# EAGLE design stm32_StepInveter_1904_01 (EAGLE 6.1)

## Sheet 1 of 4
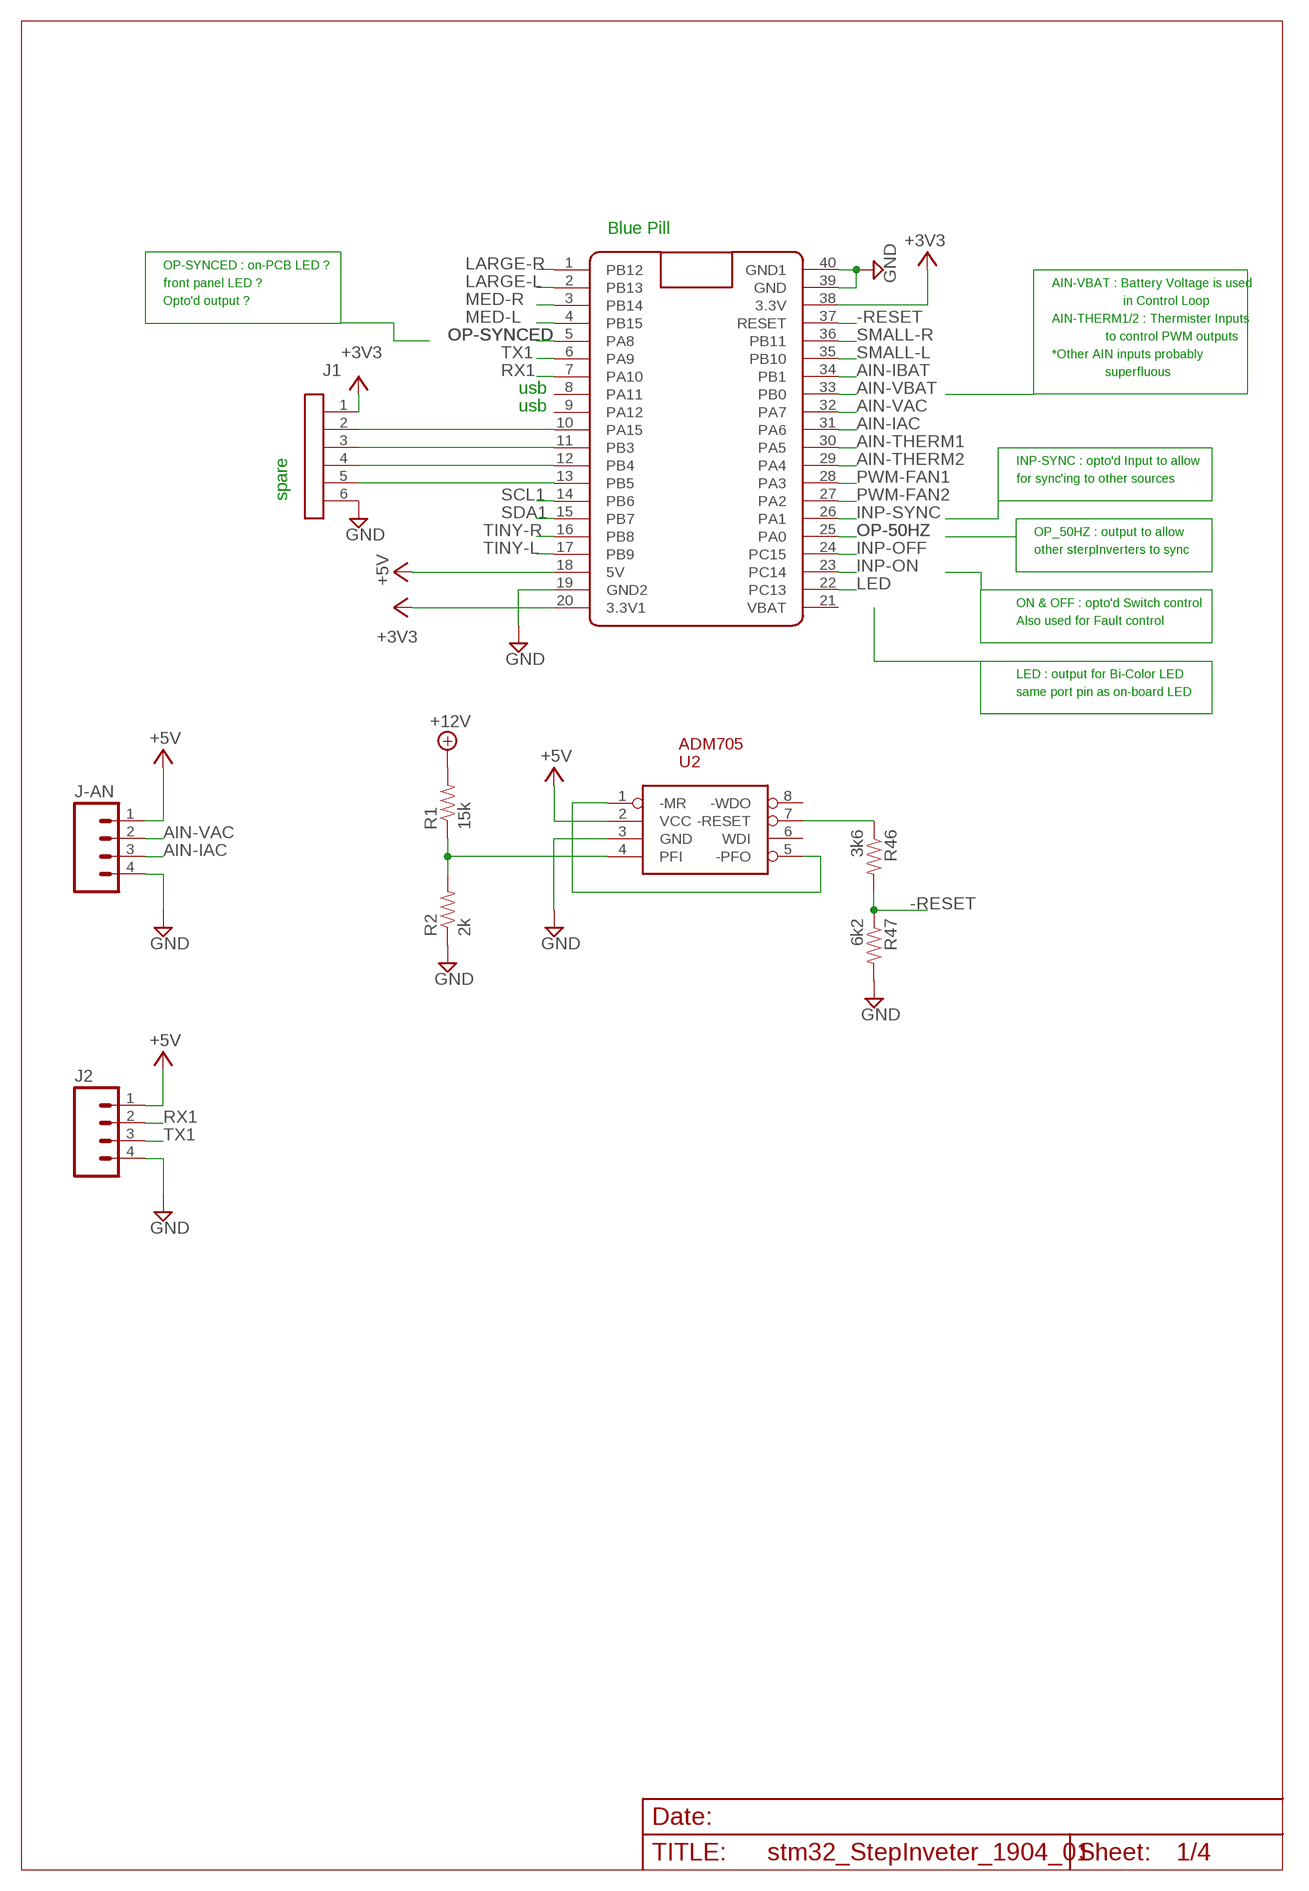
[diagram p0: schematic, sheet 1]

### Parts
J1  SIL-6  [SIL6]
J2  SIL4  [SIL4]
J-AN  SIL4  [SIL4]
R1  15k  R4  [AXIAL-0.4]
R2  2k  R4  [AXIAL-0.4]
R46  3k6  R4  [AXIAL-0.4]
R47  6k2  R4  [AXIAL-0.4]
U2  ADM705  [DIL08]
U$1  BLUE_PILL  [BLUE_PILL_CLEAN]

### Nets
+3V3: J1.1 U$1.20(3.3V1) U$1.38(3.3V) ; also sheet 3
+5V: J2.1 J-AN.1 U2.2(VCC) U$1.18(5V) ; also sheet 2,3,4
+12V: R1.P$2 ; also sheet 3
-RESET: R46.P$2 R47.P$1 U$1.37(RESET)
AIN-IAC: J-AN.3 U$1.31(PA6)
AIN-IBAT: U$1.34(PB1) ; also sheet 3
AIN-THERM1: U$1.30(PA5) ; also sheet 3
AIN-THERM2: U$1.29(PA4) ; also sheet 3
AIN-VAC: J-AN.2 U$1.32(PA7)
AIN-VBAT: U$1.33(PB0) ; also sheet 3
GND: J1.6 J2.4 J-AN.4 R2.P$1 R47.P$2 U2.3(GND) U$1.19(GND2) U$1.39(GND) U$1.40(GND1) ; also sheet 2,3,4
INP-OFF: U$1.24(PC15) ; also sheet 3
INP-ON: U$1.23(PC14) ; also sheet 3
INP-SYNC: U$1.26(PA1) ; also sheet 3
LARGE-L: U$1.2(PB13) ; also sheet 2
LARGE-R: U$1.1(PB12) ; also sheet 2
LED: U$1.22(PC13) ; also sheet 4
MED-L: U$1.4(PB15) ; also sheet 2
MED-R: U$1.3(PB14) ; also sheet 2
N$1: J1.2 U$1.10(PA15)
N$2: J1.3 U$1.11(PB3)
N$3: J1.4 U$1.12(PB4)
N$4: J1.5 U$1.13(PB5)
N$5: U2.1(-MR) U2.5(-PFO)
N$6: R1.P$1 R2.P$2 U2.4(PFI)
N$77: R46.P$1 U2.7(-RESET)
OP-50HZ: U$1.25(PA0) ; also sheet 4
OP-SYNCED: U$1.5(PA8) ; also sheet 4
PWM-FAN1: U$1.28(PA3) ; also sheet 4
PWM-FAN2: U$1.27(PA2) ; also sheet 4
RX1: J2.2 U$1.7(PA10)
SCL1: U$1.14(PB6)
SDA1: U$1.15(PB7)
SMALL-L: U$1.35(PB10) ; also sheet 2
SMALL-R: U$1.36(PB11) ; also sheet 2
TINY-L: U$1.17(PB9) ; also sheet 2
TINY-R: U$1.16(PB8) ; also sheet 2
TX1: J2.3 U$1.6(PA9)
Unconnected: U2.6(WDI) U2.8(-WDO) U$1.8(PA11) U$1.9(PA12) U$1.21(VBAT)

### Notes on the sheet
- Blue Pill
- OP-SYNCED : on-PCB LED ?
- front panel LED ? | AIN-VBAT : Battery Voltage is used
- Opto'd output ? | in Control Loop
- AIN-THERM1/2 : Thermister Inputs
- to control PWM outputs
- *Other AIN inputs probably
- superfluous
- usb
- usb
- INP-SYNC : opto'd Input to allow
- for sync'ing to other sources
- spare
- OP_50HZ : output to allow
- other sterpInverters to sync
- ON & OFF : opto'd Switch control
- Also used for Fault control
- LED : output for Bi-Color LED
- same port pin as on-board LED

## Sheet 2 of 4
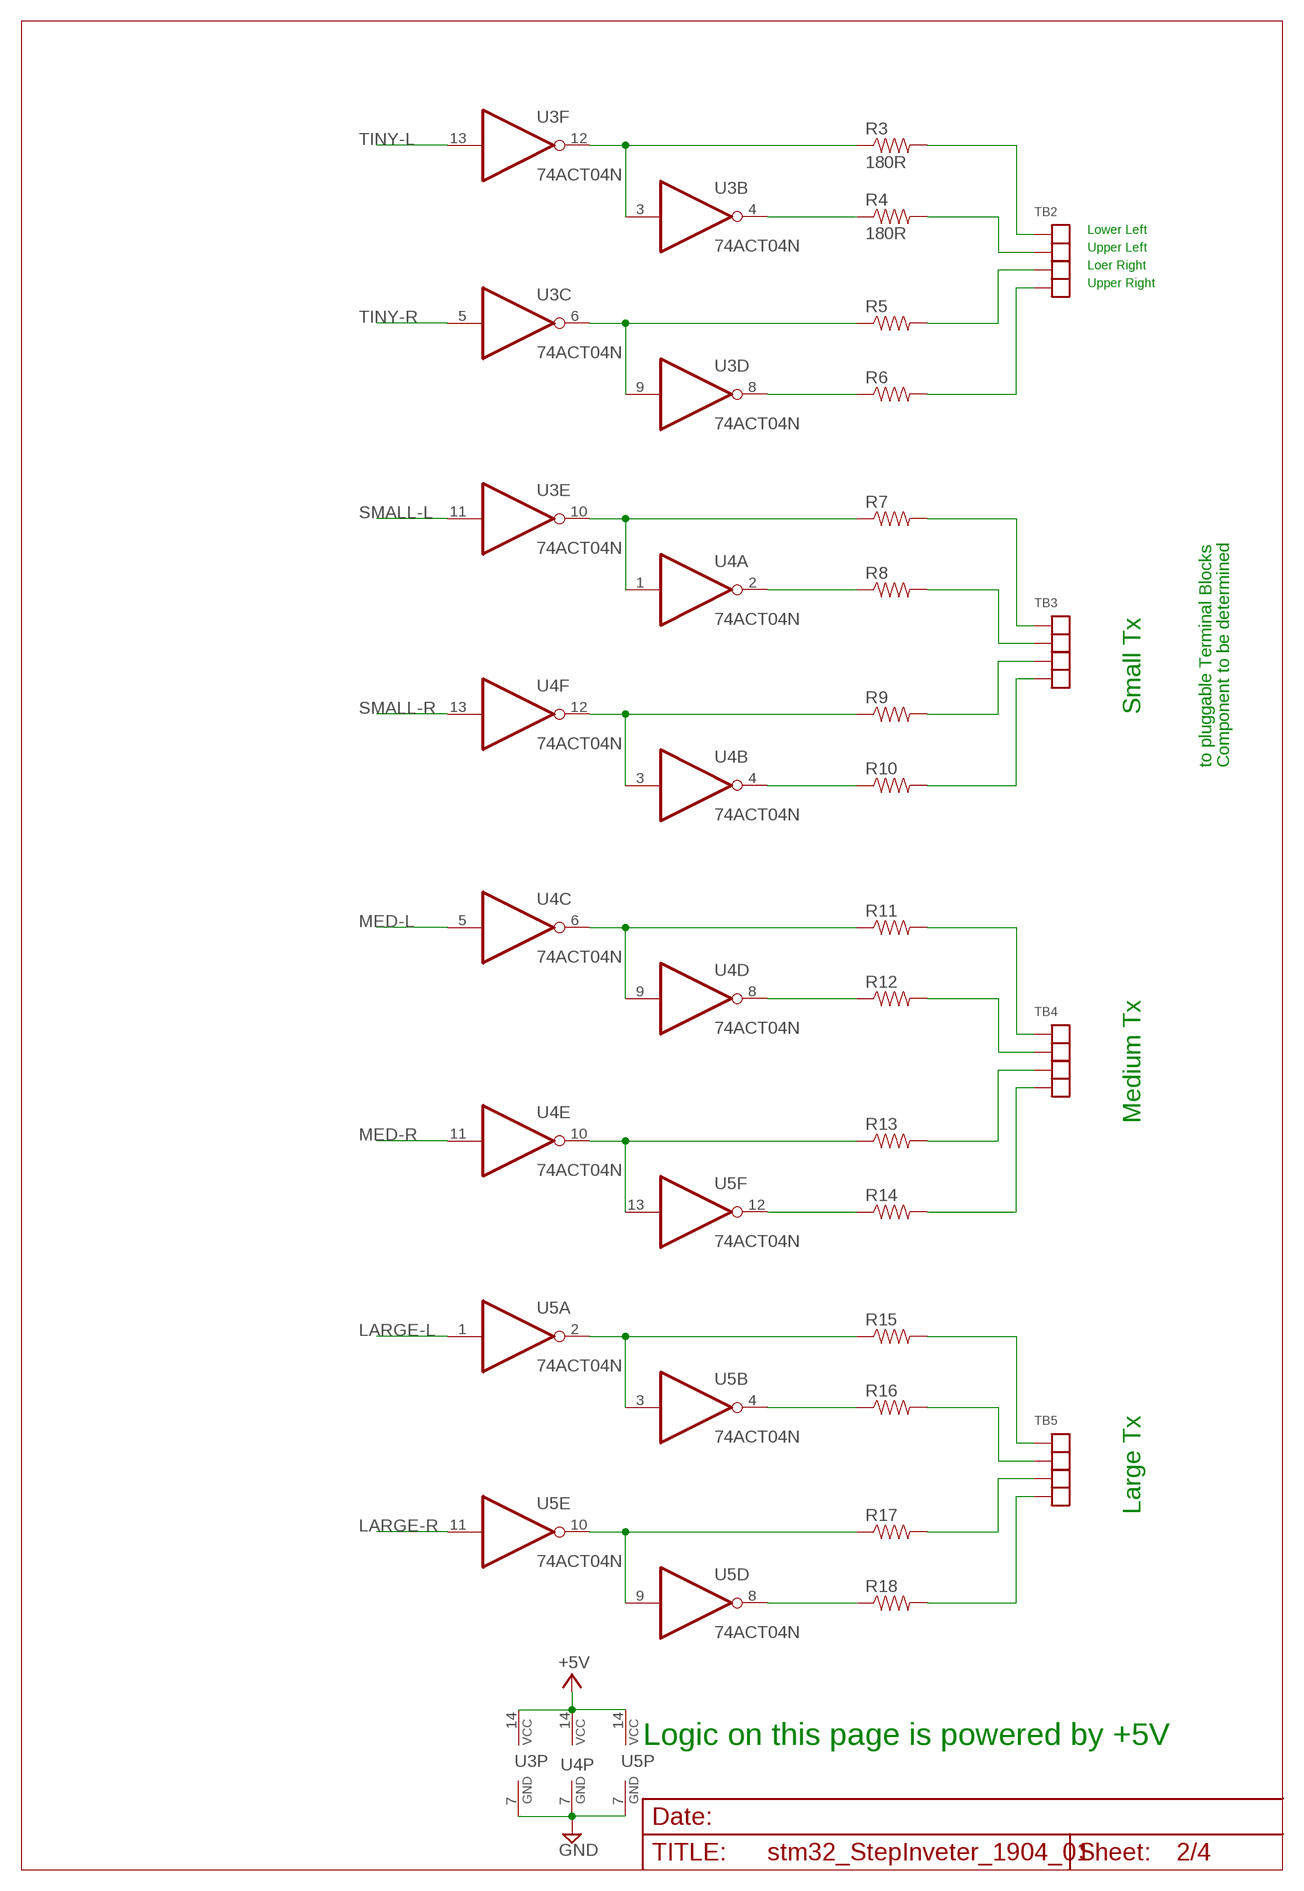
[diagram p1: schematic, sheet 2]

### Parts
R3  180R  R4  [AXIAL-0.4]
R4  180R  R4  [AXIAL-0.4]
R5  R4  [AXIAL-0.4]
R6  R4  [AXIAL-0.4]
R7  R4  [AXIAL-0.4]
R8  R4  [AXIAL-0.4]
R9  R4  [AXIAL-0.4]
R10  R4  [AXIAL-0.4]
R11  R4  [AXIAL-0.4]
R12  R4  [AXIAL-0.4]
R13  R4  [AXIAL-0.4]
R14  R4  [AXIAL-0.4]
R15  R4  [AXIAL-0.4]
R16  R4  [AXIAL-0.4]
R17  R4  [AXIAL-0.4]
R18  R4  [AXIAL-0.4]
TB2  TB4381_SIL  [TB-381-SIL-4P]
TB3  TB4381_SIL  [TB-381-SIL-4P]
TB4  TB4381_SIL  [TB-381-SIL-4P]
TB5  TB4381_SIL  [TB-381-SIL-4P]
U3  74ACT04N  [DIL14]
U4  74ACT04N  [DIL14]
U5  74ACT04N  [DIL14]

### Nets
+5V: U3.14(P:VCC) U4.14(P:VCC) U5.14(P:VCC) ; also sheet 1,3,4
GND: U3.7(P:GND) U4.7(P:GND) U5.7(P:GND) ; also sheet 1,3,4
LARGE-L: U5.1(A:I) ; also sheet 1
LARGE-R: U5.11(E:I) ; also sheet 1
MED-L: U4.5(C:I) ; also sheet 1
MED-R: U4.11(E:I) ; also sheet 1
N$15: R3.P$1 U3.3(B:I) U3.12(F:O)
N$16: R4.P$1 U3.4(B:O)
N$17: R5.P$1 U3.6(C:O) U3.9(D:I)
N$18: R6.P$1 U3.8(D:O)
N$19: R7.P$1 U3.10(E:O) U4.1(A:I)
N$20: R8.P$1 U4.2(A:O)
N$21: R9.P$1 U4.3(B:I) U4.12(F:O)
N$22: R10.P$1 U4.4(B:O)
N$23: R11.P$1 U4.6(C:O) U4.9(D:I)
N$24: R12.P$1 U4.8(D:O)
N$25: R13.P$1 U4.10(E:O) U5.13(F:I)
N$26: R14.P$1 U5.12(F:O)
N$27: R15.P$1 U5.2(A:O) U5.3(B:I)
N$28: R16.P$1 U5.4(B:O)
N$29: R17.P$1 U5.9(D:I) U5.10(E:O)
N$30: R18.P$1 U5.8(D:O)
N$40: R3.P$2 TB2.1 TB2.11
N$62: R4.P$2 TB2.2 TB2.12
N$63: R5.P$2 TB2.3 TB2.13
N$64: R6.P$2 TB2.4 TB2.14
N$65: R7.P$2 TB3.1 TB3.11
N$66: R8.P$2 TB3.2 TB3.12
N$67: R9.P$2 TB3.3 TB3.13
N$68: R10.P$2 TB3.4 TB3.14
N$69: R11.P$2 TB4.1 TB4.11
N$70: R12.P$2 TB4.2 TB4.12
N$71: R13.P$2 TB4.3 TB4.13
N$72: R14.P$2 TB4.4 TB4.14
N$73: R15.P$2 TB5.1 TB5.11
N$74: R16.P$2 TB5.2 TB5.12
N$75: R17.P$2 TB5.3 TB5.13
N$76: R18.P$2 TB5.4 TB5.14
SMALL-L: U3.11(E:I) ; also sheet 1
SMALL-R: U4.13(F:I) ; also sheet 1
TINY-L: U3.13(F:I) ; also sheet 1
TINY-R: U3.5(C:I) ; also sheet 1

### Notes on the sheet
- Lower Left
- Upper Left
- Loer Right
- Upper Right
- Small Tx
- to pluggable Terminal Blocks | Component to be determined
- Medium Tx
- Large Tx
- Logic on this page is powered by +5V

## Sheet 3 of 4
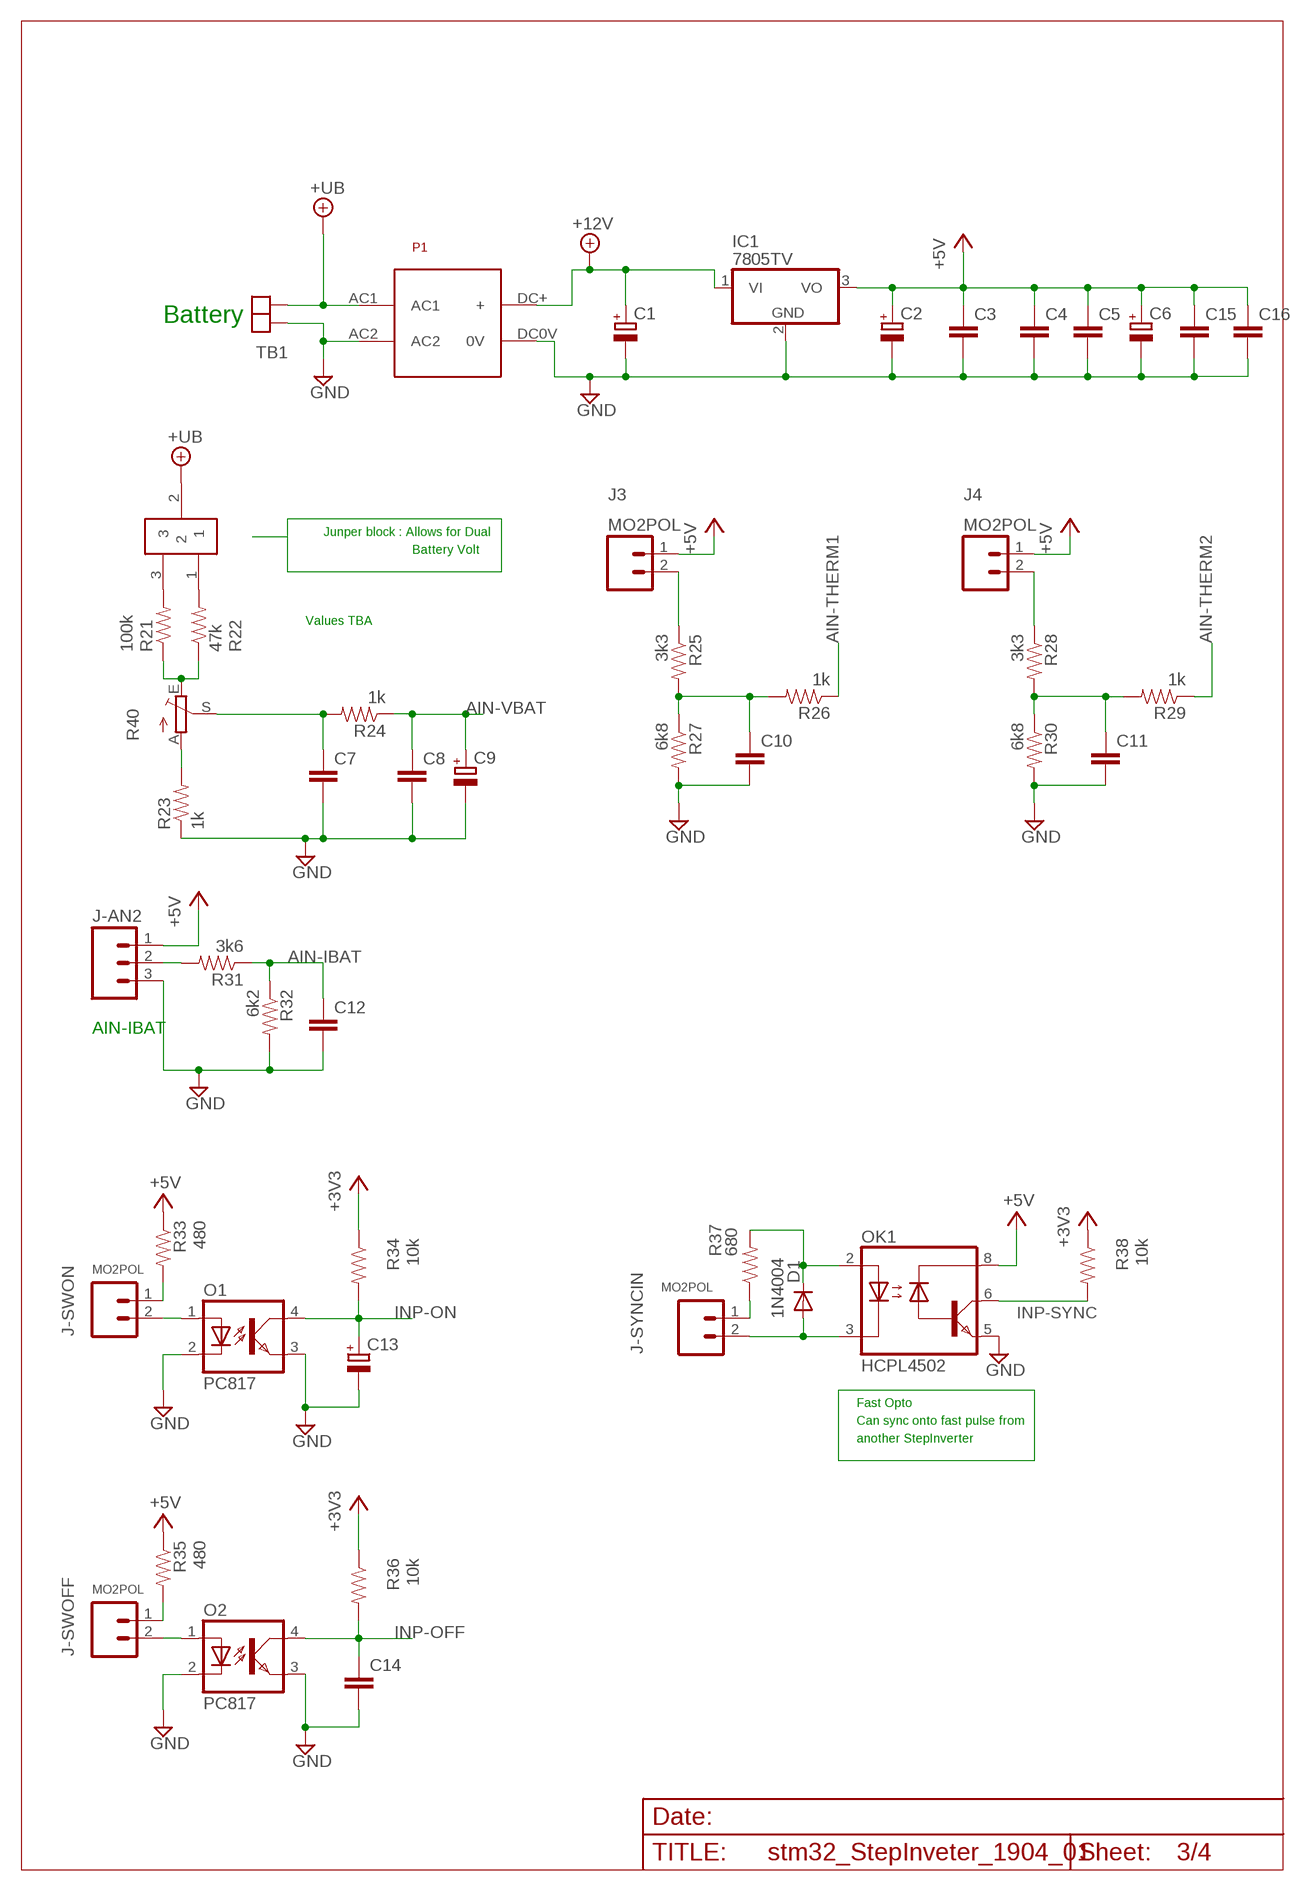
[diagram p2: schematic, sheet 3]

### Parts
C1  CPOL-EUE5-8.5  [E5-8,5]
C2  CPOL-EUE2.5-5  [E2,5-5]
C3  BCAP  [BCAP]
C4  BCAP  [BCAP]
C5  BCAP  [BCAP]
C6  CPOL-EUE2.5-5  [E2,5-5]
C7  BCAP  [BCAP]
C8  BCAP  [BCAP]
C9  CPOL-EUE2.5-5  [E2,5-5]
C10  BCAP  [BCAP]
C11  BCAP  [BCAP]
C12  BCAP  [BCAP]
C13  CPOL-EUE2.5-6  [E2,5-6]
C14  BCAP  [BCAP]
C15  BCAP  [BCAP]
C16  BCAP  [BCAP]
D1  1N4004  [DO41-10]
IC1  7805TV  [TO220V]
J3  MO2POL  [MOLEX-1X2]
J4  MO2POL  [MOLEX-1X2]
J-AN2  MO3POL  [MOLEX-3]
J-SWOFF  MO2POL  [MOLEX-1X2]
J-SWON  MO2POL  [MOLEX-1X2]
J-SYNCIN  MO2POL  [MOLEX-1X2]
JP1  JP1X3  [JP1X3]
O1  PC817  [DIL04]
O2  PC817  [DIL04]
OK1  HCPL4502  [DIL08]
P1  ACDC  [ACDC]
R21  100k  R4  [AXIAL-0.4]
R22  47k  R4  [AXIAL-0.4]
R23  1k  R4  [AXIAL-0.4]
R24  1k  R4  [AXIAL-0.4]
R25  3k3  R4  [AXIAL-0.4]
R26  1k  R4  [AXIAL-0.4]
R27  6k8  R4  [AXIAL-0.4]
R28  3k3  R4  [AXIAL-0.4]
R29  1k  R4  [AXIAL-0.4]
R30  6k8  R4  [AXIAL-0.4]
R31  3k6  R4  [AXIAL-0.4]
R32  6k2  R4  [AXIAL-0.4]
R33  480  R4  [AXIAL-0.4]
R34  10k  R4  [AXIAL-0.4]
R35  480  R4  [AXIAL-0.4]
R36  10k  R4  [AXIAL-0.4]
R37  680  R4  [AXIAL-0.4]
R38  10k  R4  [AXIAL-0.4]
R40  TRIM_EU-B64Y  [B64Y]
TB1  TB2381  [TB-KF2EDG381-2P]

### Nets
+3V3: R34.P$1 R36.P$1 R38.P$1 ; also sheet 1
+5V: C2.+ C3.1 C4.1 C5.1 C6.+ C15.1 C16.1 IC1.3(VO) J3.1 J4.1 J-AN2.1 OK1.8(VCC) R33.P$1 R35.P$1 ; also sheet 1,2,4
+12V: C1.+ IC1.1(VI) P1.DC+(+) ; also sheet 1
+UB: JP1.2 P1.AC1 TB1.1
AIN-IBAT: C12.1 R31.P$1 R32.P$1 ; also sheet 1
AIN-THERM1: R26.P$1 ; also sheet 1
AIN-THERM2: R29.P$1 ; also sheet 1
AIN-VBAT: C8.1 C9.+ R24.P$1 ; also sheet 1
GND: C1.- C2.- C3.2 C4.2 C5.2 C6.- C7.2 C8.2 C9.- C10.2 C11.2 C12.2 C13.- C14.2 C15.2 C16.2 IC1.2(GND) J-AN2.3 O1.2(C) O1.3(EMIT) O2.2(C) O2.3(EMIT) OK1.5(GND) P1.AC2 P1.DC0V(0V) R23.P$1 R27.P$2 R30.P$2 R32.P$2 TB1.2 ; also sheet 1,2,4
INP-OFF: C14.1 O2.4(COL) R36.P$2 ; also sheet 1
INP-ON: C13.+ O1.4(COL) R34.P$2 ; also sheet 1
INP-SYNC: OK1.6(VO) R38.P$2 ; also sheet 1
N$14: JP1.3 R21.P$2
N$32: JP1.1 R22.P$2
N$34: R21.P$1 R22.P$1 R40.E
N$35: C10.1 R25.P$2 R26.P$2 R27.P$1
N$36: J4.2 R28.P$1
N$37: J3.2 R25.P$1
N$38: C11.1 R28.P$2 R29.P$2 R30.P$1
N$39: J-SWON.1 R33.P$2
N$41: J-AN2.2 R31.P$2
N$42: J-SWON.2 O1.1(A)
N$43: J-SYNCIN.1 R37.P$1
N$44: D1.A J-SYNCIN.2 OK1.3(C)
N$45: J-SWOFF.1 R35.P$2
N$46: J-SWOFF.2 O2.1(A)
N$47: D1.C OK1.2(A) R37.P$2
N$82: C7.1 R24.P$2 R40.S
N$84: R23.P$2 R40.A

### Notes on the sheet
- Battery
- Junper block : Allows for Dual
- Battery Volt
- Values TBA
- AIN-IBAT
- Fast Opto
- Can sync onto fast pulse from
- another StepInverter

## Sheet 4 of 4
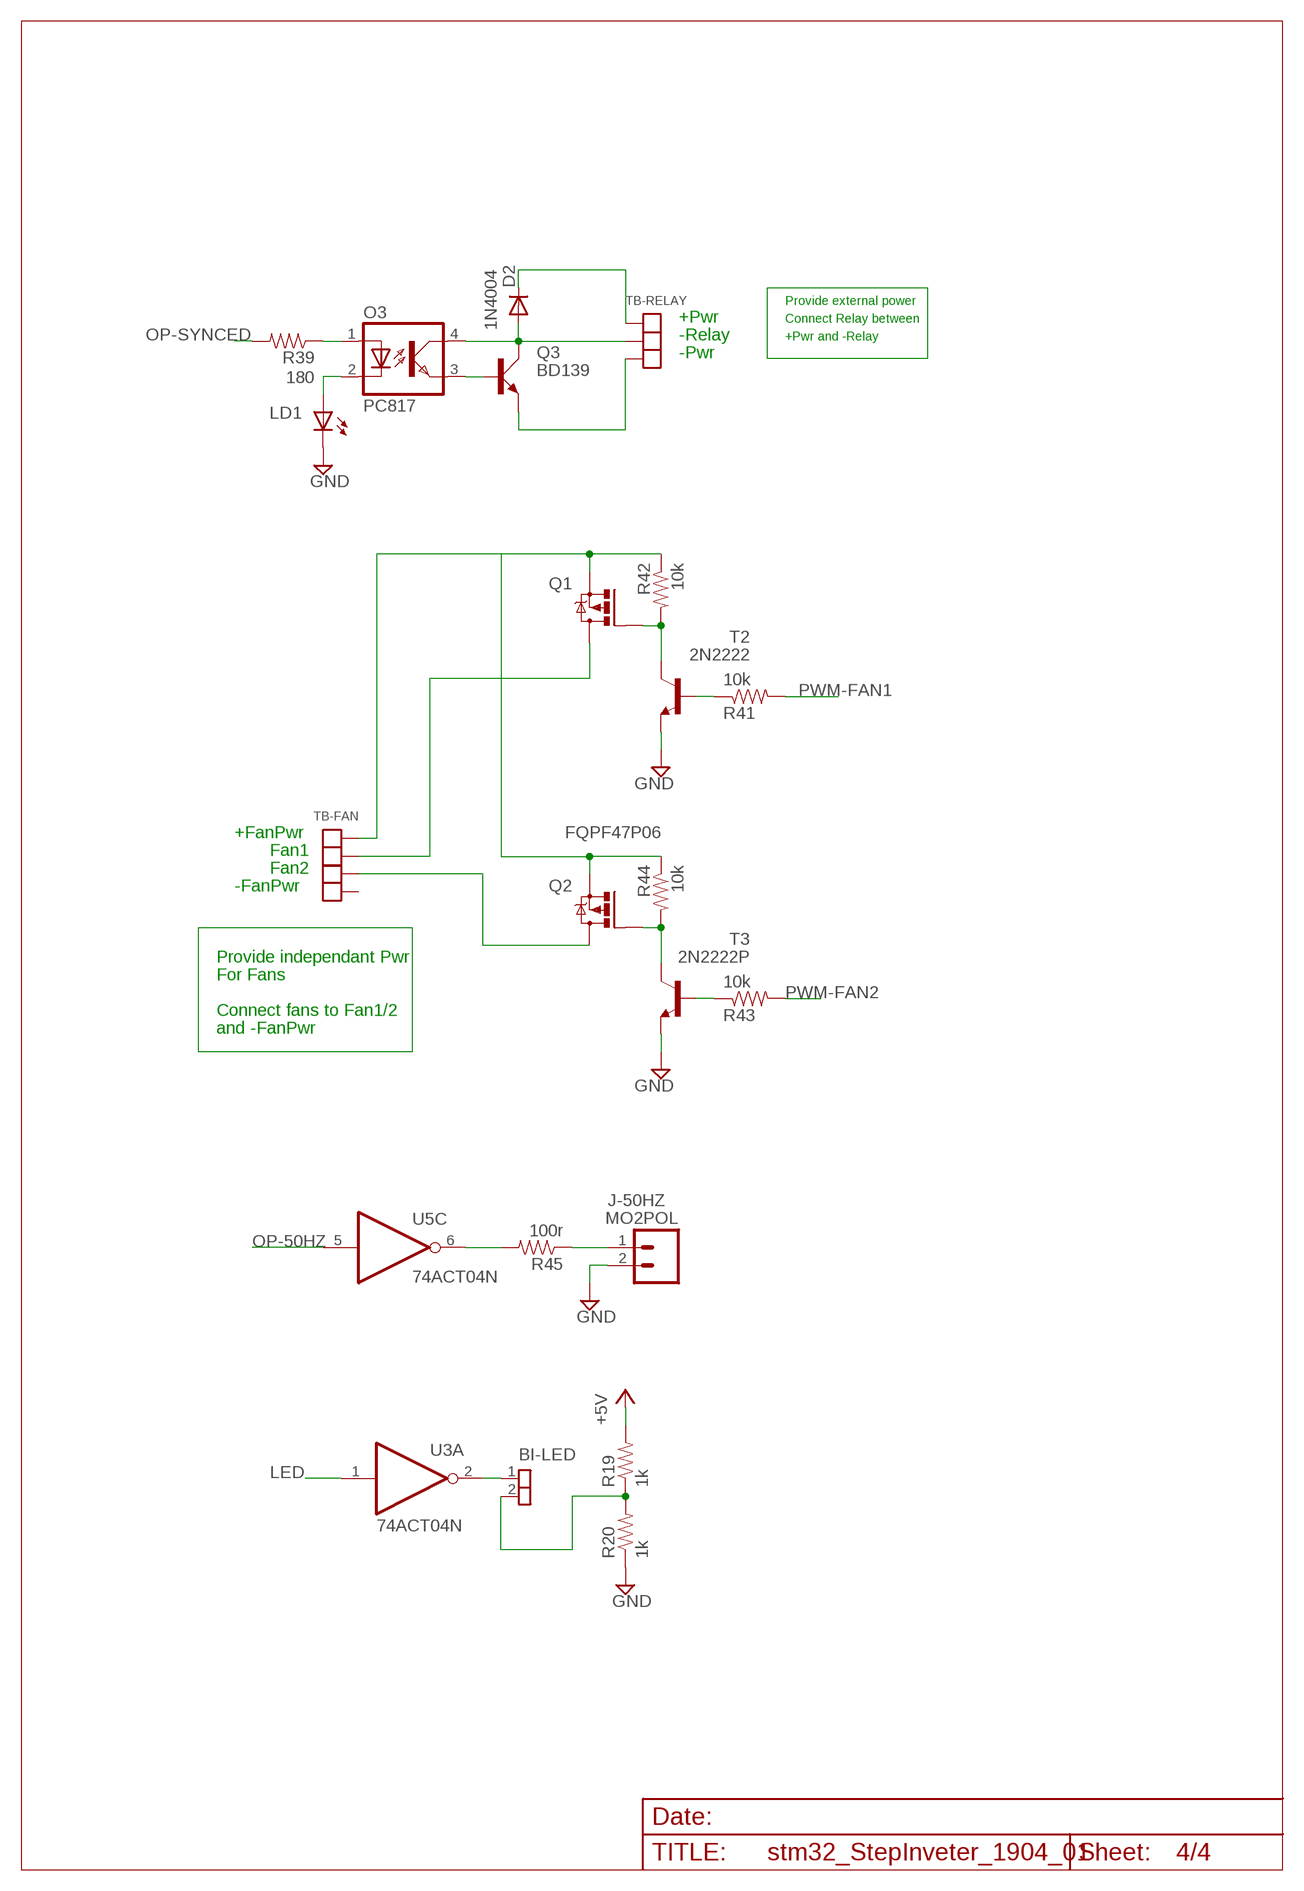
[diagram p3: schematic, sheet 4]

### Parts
BI-LED  SIL-2  [JP1]
D2  1N4004  [DO41-10]
J-50HZ  MO2POL  [MOLEX-1X2]
LD1  LED3MM  [LED3MM]
O3  PC817  [DIL04]
Q1  MOSFET-PCHFQPF47P06  [TO220BV]
Q2  FQPF47P06  MOSFET-PCHFQPF47P06  [TO220BV]
Q3  BD139  [TO126AV]
R19  1k  R4  [AXIAL-0.4]
R20  1k  R4  [AXIAL-0.4]
R39  180  R4  [AXIAL-0.4]
R41  10k  R4  [AXIAL-0.4]
R42  10k  R4  [AXIAL-0.4]
R43  10k  R4  [AXIAL-0.4]
R44  10k  R4  [AXIAL-0.4]
R45  100r  R4  [AXIAL-0.4]
T2  2N2222  2N2222P  [TO92/]
T3  2N2222P  [TO92/]
TB-FAN  TB4  [TB-KF2EDG381-4P]
TB-RELAY  TB3381  [TB-KF2EDG381-3P]

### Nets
+5V: R19.P$2 ; also sheet 1,2,3
GND: J-50HZ.2 LD1.K(C) R20.P$1 T2.1(E) T3.1(E) ; also sheet 1,2,3
LED: U3.1(A:I) ; also sheet 1
N$7: BI-LED.2 R19.P$1 R20.P$2
N$8: BI-LED.1 U3.2(A:O)
N$49: LD1.A O3.2(C)
N$50: O3.1(A) R39.P$1
N$51: Q1.G R42.P$2 T2.3(C)
N$52: O3.3(EMIT) Q3.B
N$53: R41.P$1 T2.2(B)
N$54: Q1.S Q2.S R42.P$1 R44.P$1 TB-FAN.1
N$55: Q2.G R44.P$2 T3.3(C)
N$56: R45.P$2 U5.6(C:O)
N$57: Q1.D TB-FAN.2
N$58: R43.P$1 T3.2(B)
N$59: J-50HZ.1 R45.P$1
N$60: Q2.D TB-FAN.3
N$78: D2.A O3.4(COL) Q3.C TB-RELAY.2
N$79: D2.C TB-RELAY.1
N$81: Q3.E TB-RELAY.3
OP-50HZ: U5.5(C:I) ; also sheet 1
OP-SYNCED: R39.P$2 ; also sheet 1
PWM-FAN1: R41.P$2 ; also sheet 1
PWM-FAN2: R43.P$2 ; also sheet 1
Unconnected: TB-FAN.4

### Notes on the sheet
- Provide external power
- +Pwr | Connect Relay between
- -Relay | +Pwr and -Relay
- -Pwr
- +FanPwr
- Fan1
- Fan2
- -FanPwr
- Provide independant Pwr
- For Fans
- Connect fans to Fan1/2
- and -FanPwr

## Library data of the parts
BI-LED = Andrew_Connectors:SIL-2
C1 C2 C6 C9 C13 = rcl:CPOL-EU: POLARIZED CAPACITOR, European symbol
C3-C5 C7 C8 C10-C12 C14-C16 = Andrew Misc:BCAP
D1 D2 = diode:1N4004: DIODE
IC1 = Andrew Linear:78*: Positive VOLTAGE REGULATOR Source: http://cache.national.com/ds/LM/LM78L05.pdf http://www.fairchildsemi.com/ds/LM/LM7805.pdf
J1 = Andrew_Connectors:SIL-6
J2 J-AN = Andrew_Connectors:SIL4
J3 J4 J-50HZ J-SWOFF J-SWON J-SYNCIN = Andrew_Connectors:MO2POL
J-AN2 = Andrew_Connectors:MO3POL
JP1 = Andrew_Connectors:JP1X3
LD1 = led:LED: LED
O1-O3 = Andrew:PC817: SHARP OPTO COUPLER; MPN: PC817X4J000F; OC_FARNELL: 9707727; OC_NEWARK: 97K7059
OK1 = optocoupler:HCPL4502: HEWLETT PACKARD OPTO COUPLER; MF: AGILENT TECHNOLOGIES; MPN: HCPL-4502-000E; OC_FARNELL: 9994777; OC_NEWARK: 31K7017
P1 = Andrew ISOPWR:ACDC
Q1 Q2 = Andrew Transistor:MOSFET-PCH: P-CHANNEL HEXFET POWER-MOS-FET Source: http://www.irf.com/product-info/datasheets/data/irf9530.pdf
Q3 = transistor-power:BD139: NPN TRANSISTOR
R1-R39 R41-R47 = Andrew Misc:R4
R40 = pot:TRIM_EU-: POTENTIOMETER
T2 T3 = Andrew Transistor:2N2222: NPN TRANSISTOR
TB1 = Andrew_Connectors:TB2
TB2-TB5 TB-FAN = Andrew_Connectors:TB4
TB-RELAY = Andrew_Connectors:TB3
U2 = Andrew IC:ADM705
U3-U5 = 74xx-eu:74*04: Hex INVERTER
U$1 = Andrew_BluePill_Scope:BLUE_PILL

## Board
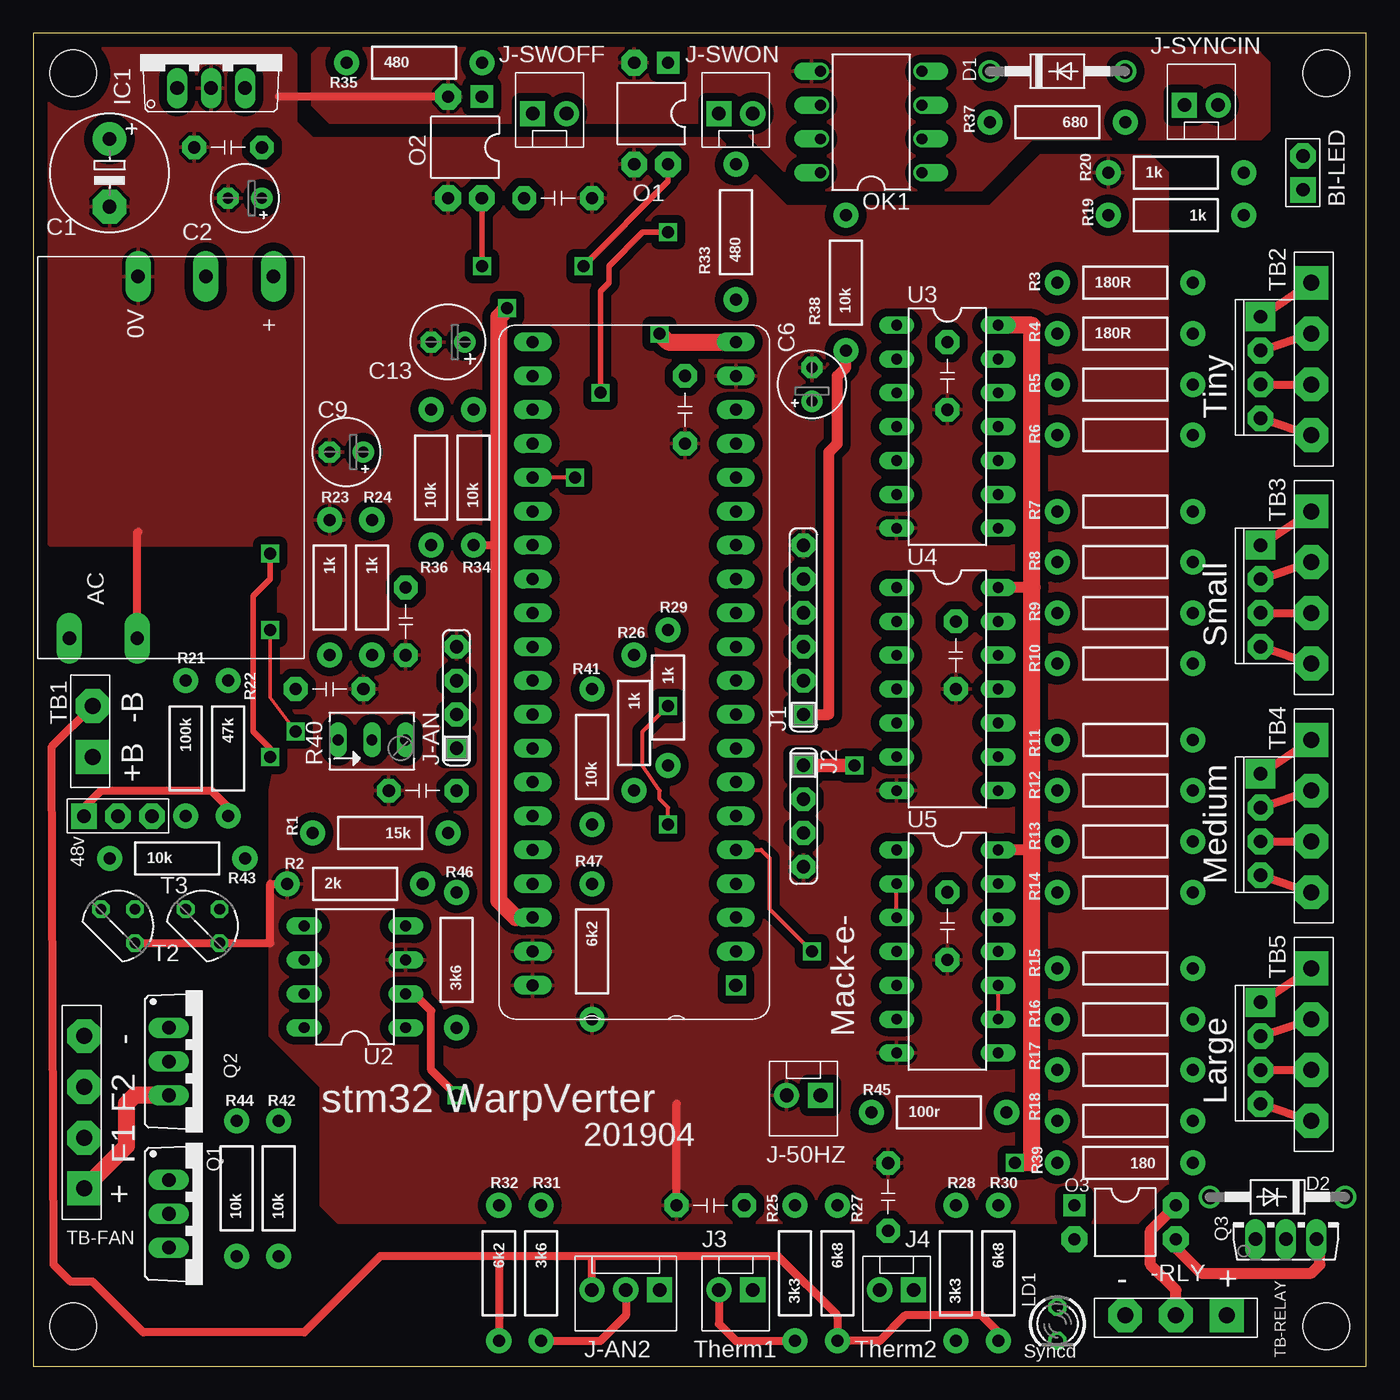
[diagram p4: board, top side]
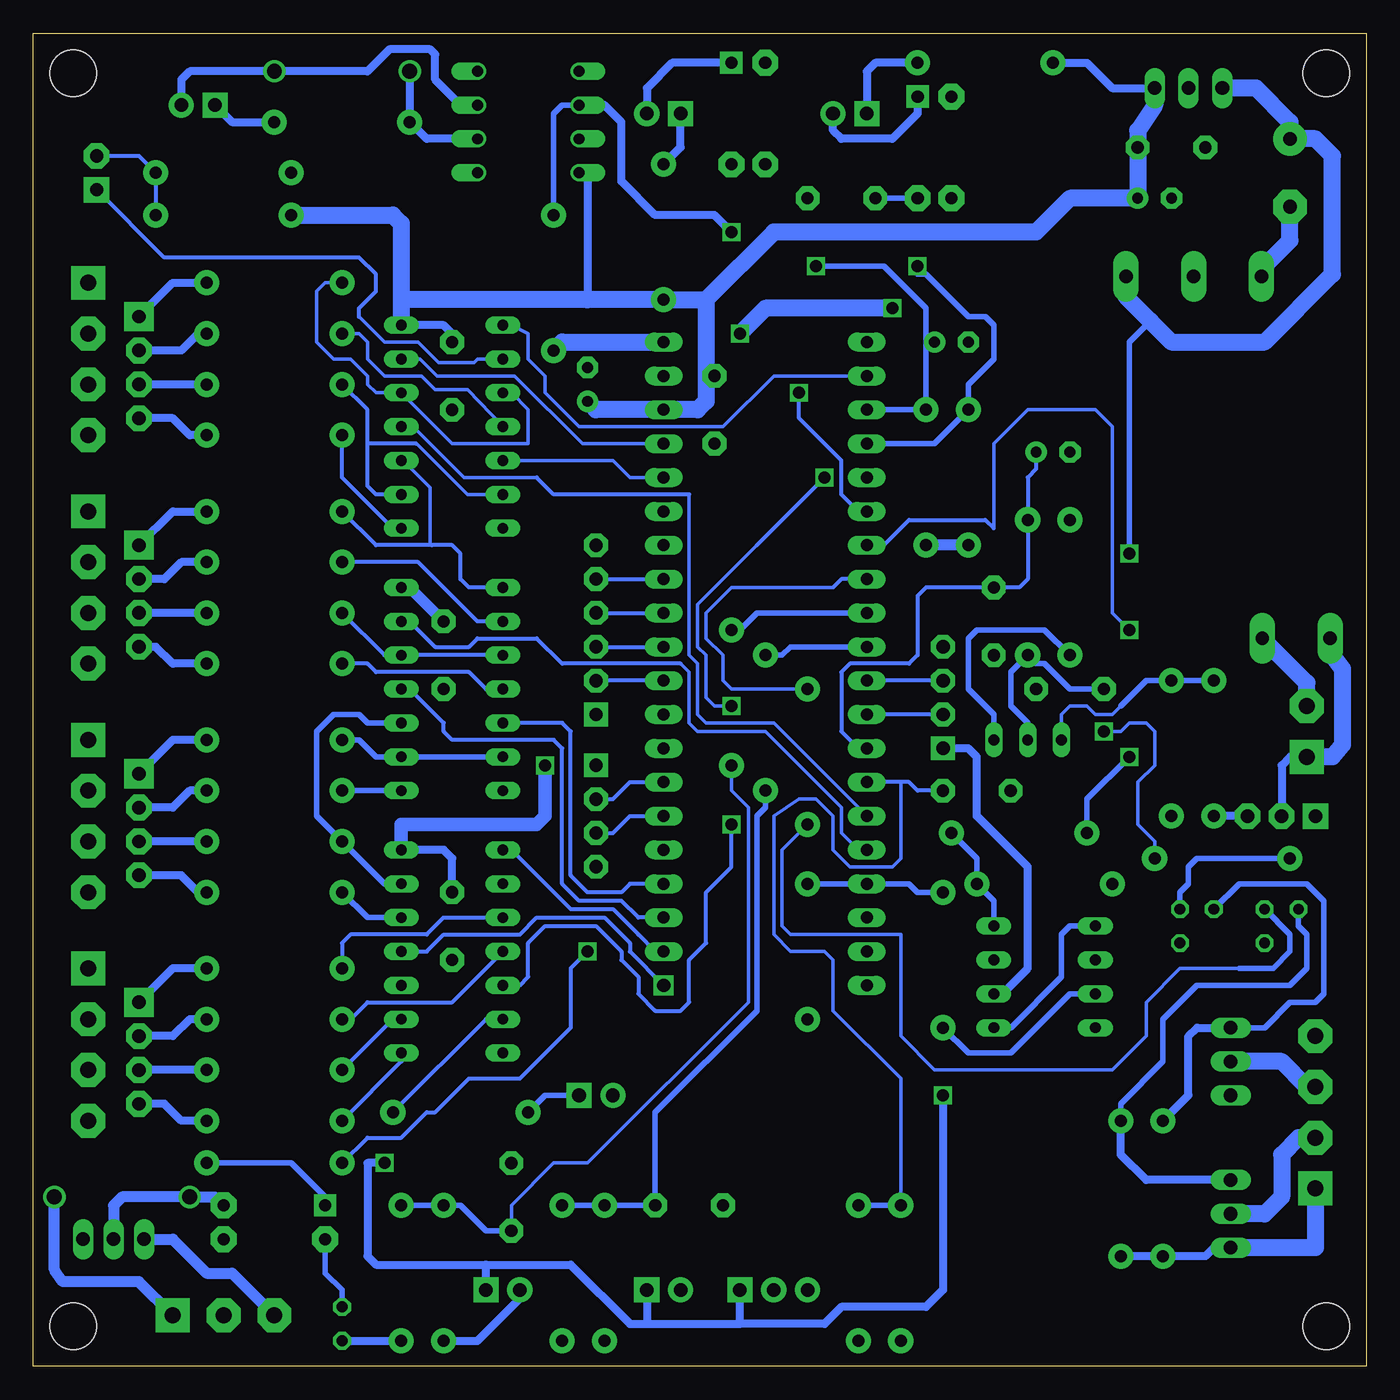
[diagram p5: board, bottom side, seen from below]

Size 100 x 100 mm. Coordinates in mm from the lower left corner, seen from the top.
Outline: 0,0 100,0 100,100 0,100 0,0
Copper layers (1*16): Top 0.035mm / dielectric 1.5mm / Bottom 0.035mm
Design rules: minimum track width 10mil, minimum drill 24mil, track to track 8mil, track to pad 8mil, pad to pad 8mil, via to via 8mil, smd to smd 8mil, copper to edge 40mil, drill to drill 8mil, minimum pad ring 10mil, minimum via ring 8mil, stop-mask expansion 4mil, vias tented up to drill 0mil, thermal gap 10mil
Holes 3.5 mm at 3,3 3,97 97,97 97,3

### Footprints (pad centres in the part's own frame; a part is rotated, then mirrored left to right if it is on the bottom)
JP1 = drill 1 pad 1.905 square: 1 -1.27,0 | drill 1 pad 1.905 octagon: 2 1.27,0
E5-8,5 = drill 1.016 pad 2.54: + -2.54,0 | drill 1.016 pad 2.54 octagon: - 2.54,0
E2,5-5 = drill 0.813 pad 1.6: + -1.27,0 | drill 0.813 pad 1.6 octagon: - 1.27,0
BCAP = drill 0.914 pad 1.778 octagon: 1 -2.54,0; 2 2.54,0
E2,5-6 = drill 0.813 pad 1.6: + -1.27,0 | drill 0.813 pad 1.6 octagon: - 1.27,0
DO41-10 = drill 1.118: A 5.08,0; C -5.08,0
TO220V = drill 1.016 long: 1 -2.54,-2.54; 2 0,-2.54; 3 2.54,-2.54
SIL6 = drill 1 pad 1.778 square: 1 -6.35,0 | drill 1 pad 1.778 octagon: 2 -3.81,0; 3 -1.27,0; 4 1.27,0; 5 3.81,0; 6 6.35,0
SIL4 = drill 1 pad 1.778 square: 1 0,0 | drill 1 pad 1.778 octagon: 2 2.54,0; 3 5.08,0; 4 7.62,0
MOLEX-1X2 = drill 1.016 pad 1.88 square: 1 0,0 | drill 1.016 pad 1.88: 2 2.54,0
MOLEX-3 = drill 1.016 pad 1.88 square: 1 -2.54,0 | drill 1.016 pad 1.88: 2 0,0; 3 2.54,0
JP1X3 = drill 1 pad 1.905 square: 1 -2.54,0 | drill 1 pad 1.905 octagon: 2 0,0; 3 2.54,0
LED3MM = drill 0.813 octagon: A -1.27,0; K 1.27,0
DIL04 = drill 0.914 pad 1.676 square: 1 -1.27,-3.81 | drill 0.914 pad 1.93 octagon: 2 1.27,-3.81; 3 1.27,3.81; 4 -1.27,3.81
DIL08 = drill 0.813 offset: 1 -3.81,-3.81; 2 -1.27,-3.81; 3 1.27,-3.81; 4 3.81,-3.81; 5 3.81,3.81; 6 1.27,3.81; 7 -1.27,3.81; 8 -3.81,3.81
ACDC = drill 1 pad 1.93 long: 4 27.15,7.38; AC1 0,17.61; AC2 0,12.53; DC0V 27.15,12.46; DC+ 27.15,2.3
TO220BV = drill 1.016 long: D 0,-2.54; G -2.54,-2.54; S 2.54,-2.54
TO126AV = drill 1.016 long: B 2.286,-1.27; C 0,-1.27; E -2.286,-1.27
AXIAL-0.4 = drill 0.9 pad 1.88: P$1 -5.08,0; P$2 5.08,0
B64Y = drill 0.813 long: A 2.54,0; E -2.54,0; S 0,0
TO92/ = drill 0.813 octagon: 1 1.27,-1.27; 2 1.27,1.27; 3 -1.27,1.27
TB-KF2EDG381-2P = drill 1.2 pad 2.54 square: 1 0,0 | drill 1.2 pad 2.54 octagon: 2 3.81,0
TB-381-SIL-4P = drill 1.2 pad 2.54 square: 1 0,0 | drill 1.2 pad 2.54 octagon: 2 3.81,0; 3 7.62,0; 4 11.43,0 | drill 1 pad 2.184 square: 11 2.54,-3.81 | drill 1 pad 1.93 octagon: 12 5.08,-3.81; 13 7.62,-3.81; 14 10.16,-3.81
TB-KF2EDG381-4P = drill 1.2 pad 2.54 square: 1 0,0 | drill 1.2 pad 2.54 octagon: 2 3.81,0; 3 7.62,0; 4 11.43,0
TB-KF2EDG381-3P = drill 1.2 pad 2.54 square: 1 0,0 | drill 1.2 pad 2.54 octagon: 2 3.81,0; 3 7.62,0
DIL08' = drill 0.813 long: 1 -3.81,-3.81; 2 -1.27,-3.81; 3 1.27,-3.81; 4 3.81,-3.81; 5 3.81,3.81; 6 1.27,3.81; 7 -1.27,3.81; 8 -3.81,3.81
DIL14 = drill 0.813 long: 1 -7.62,-3.81; 2 -5.08,-3.81; 3 -2.54,-3.81; 4 0,-3.81; 5 2.54,-3.81; 6 5.08,-3.81; 7 7.62,-3.81; 8 7.62,3.81; 9 5.08,3.81; 10 2.54,3.81; 11 0,3.81; 12 -2.54,3.81; 13 -5.08,3.81; 14 -7.62,3.81
BLUE_PILL_CLEAN = drill 1 square: 1 0,0 | drill 0.9 long: 2 0,-2.54; 3 0,-5.08; 4 0,-7.62; 5 0,-10.16; 6 0,-12.7; 7 0,-15.24; 8 0,-17.78; 9 0,-20.32; 10 0,-22.86; 11 0,-25.4; 12 0,-27.94; 13 0,-30.48; 14 0,-33.02; 15 0,-35.56; 16 0,-38.1; 17 0,-40.64; 18 0,-43.18; 19 0,-45.72; 20 0,-48.26; 21 15.24,-48.26; 22 15.24,-45.72; 23 15.24,-43.18; 24 15.24,-40.64; 25 15.24,-38.1; 26 15.24,-35.56; 27 15.24,-33.02; 28 15.24,-30.48; 29 15.24,-27.94; 30 15.24,-25.4; 31 15.24,-22.86; 32 15.24,-20.32; 33 15.24,-17.78; 34 15.24,-15.24; 35 15.24,-12.7; 36 15.24,-10.16; 37 15.24,-7.62; 38 15.24,-5.08; 39 15.24,-2.54; 40 15.24,0

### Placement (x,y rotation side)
BI-LED  95.25,89.53 90 top
C1  5.71,89.53 270 top
C2  15.88,87.63 180 top
C3  68.58,33.02 270 top
C4  14.61,91.44 180 top
C5  48.9,71.75 270 top
C6  58.42,73.66 90 top
C7  22.23,50.8 0 top
C8  27.94,55.88 270 top
C9  23.5,68.58 180 top
C10  50.8,12.06 180 top
C11  64.14,12.7 90 top
C12  29.21,43.18 180 top
C13  31.11,76.83 180 top
C14  39.37,87.63 0 top
C15  68.58,74.3 270 top
C16  69.22,53.34 270 top
D1  76.83,97.16 0 top
D2  93.34,12.7 180 top
IC1  13.34,98.42 0 top
J1  57.78,55.24 90 top
J2  57.78,45.09 270 top
J3  53.98,5.71 180 top
J4  66.04,5.71 180 top
J-50HZ  59.05,20.32 180 top
J-AN  31.75,46.35 90 top
J-AN2  44.45,5.71 180 top
J-SWOFF  37.47,93.98 0 top
J-SWON  51.44,93.98 0 top
J-SYNCIN  86.36,94.61 0 top
JP1  6.35,41.27 0 top
LD1  76.83,3.17 270 top
O1  46.35,93.98 180 top
O2  32.38,91.44 180 top
O3  81.92,10.79 270 top
OK1  62.87,93.34 90 top
P1  20.32,54.61 90 top
Q1  12.7,11.43 270 top
Q2  12.7,22.86 270 top
Q3  93.98,10.79 0 top
R1  26.04,40.01 180 top
R2  24.13,36.2 0 top
R3  81.92,81.28 0 top
R4  81.92,77.47 0 top
R5  81.92,73.66 0 top
R6  81.92,69.85 0 top
R7  81.92,64.14 0 top
R8  81.92,60.33 0 top
R9  81.92,56.52 0 top
R10  81.92,52.7 0 top
R11  81.92,46.99 0 top
R12  81.92,43.18 0 top
R13  81.92,39.37 0 top
R14  81.92,35.56 0 top
R15  81.92,29.84 0 top
R16  81.92,26.04 0 top
R17  81.92,22.23 0 top
R18  81.92,18.41 0 top
R19  85.72,86.36 180 top
R20  85.72,89.53 0 top
R21  11.43,46.35 270 top
R22  14.61,46.35 270 top
R23  22.23,58.42 270 top
R24  25.4,58.42 270 top
R25  57.15,6.99 90 top
R26  45.09,48.26 270 top
R27  60.33,6.99 270 top
R28  69.22,6.99 90 top
R29  47.62,50.16 270 top
R30  72.39,6.99 270 top
R31  38.1,6.99 270 top
R32  34.92,6.99 270 top
R33  52.7,85.09 90 top
R34  33.02,66.67 90 top
R35  28.57,97.79 0 top
R36  29.84,66.67 90 top
R37  76.83,93.34 180 top
R38  60.96,81.28 90 top
R39  81.92,15.24 180 top
R40  25.4,46.99 0 top
R41  41.91,45.72 90 top
R42  18.41,13.34 90 top
R43  10.79,38.1 0 top
R44  15.24,13.34 90 top
R45  67.94,19.05 0 top
R46  31.75,30.48 90 top
R47  41.91,31.11 270 top
T2  6.35,33.02 0 top
T3  12.7,33.02 0 top
TB1  4.45,45.72 90 top
TB2  95.89,81.28 270 top
TB3  95.89,64.14 270 top
TB4  95.89,46.99 270 top
TB5  95.89,29.84 270 top
TB-FAN  3.81,13.34 90 top
TB-RELAY  89.53,3.81 180 top
U2  ADM705  [DIL08']  24.13,29.21 90 top
U3  68.58,70.48 270 top
U4  68.58,50.8 270 top
U5  68.58,31.11 270 top
U$1  52.7,28.57 180 top

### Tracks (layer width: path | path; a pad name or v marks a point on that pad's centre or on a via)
+3V3  (via drill 0.9)
  Top 0.61: R34.P$1 34.92,61.59
  Top 0.813: J1.1 59.69,48.9 59.69,68.58 60.33,69.22 60.33,74.3 60.96,74.93 R38.P$1
  Top 1.27: U$1.38 36.2,33.66 34.92,34.92 34.92,61.59 34.92,78.74 v35.56,79.38 | v46.99,77.47 47.62,76.83 U$1.20
  Bottom 0.813: R36.P$1 R34.P$1
  Bottom 1.27: R38.P$1 60.33,76.83 U$1.20 | v35.56,79.38 45.09,79.38 v46.99,77.47
+5V  (via drill 0.9)
  Top 0.61: v31.75,20.32 29.84,22.23 29.84,26.67 28.57,27.94 U2.2
  Top 0.813: 74.93,58.42 U4.14 | 74.93,38.73 U5.14
  Top 1.016: J2.1 v61.59,45.09
  Top 1.27: U3.14 74.93,78.11 74.93,58.42 74.93,38.73 74.93,15.24 v73.66,15.24
  Bottom 0.254: 49.53,74.3 C5.1
  Bottom 0.61: OK1.8 58.42,89.53 58.42,80.01 | C15.1 68.58,77.47 69.22,78.11 U3.14 | C3.1 68.58,38.1 69.22,38.73 U5.14 | J4.1 66.04,7.62 | 66.04,7.62 59.69,7.62 55.24,3.17 53.98,3.17 | 53.98,3.17 46.99,3.17 | 46.99,3.17 J-AN2.1 | J3.1 53.98,3.17 | v73.66,15.24 74.93,15.24 74.93,8.26 74.3,7.62 66.04,7.62 | R35.P$1 20.95,97.79 19.05,95.89 IC1.3 | U2.2 27.3,27.94 25.4,29.84 25.4,37.47 29.21,41.27 29.21,45.72 29.84,46.35 J-AN.1 | v31.75,20.32 31.75,5.71 33.02,4.45 39.37,4.45 40.64,3.17 46.99,3.17
  Bottom 0.813: C16.1 71.75,58.42 U4.14
  Bottom 1.016: v61.59,45.09 61.59,41.27 62.23,40.64 72.39,40.64 U5.14
  Bottom 1.27: IC1.3 15.88,94.61 17.14,92.71 C4.1 C2.+ 22.23,87.63 24.77,85.09 44.45,85.09 49.53,80.01 | 49.53,80.01 49.53,74.3 49.53,72.39 50.16,71.75 U$1.18 57.78,71.75 C6.+ | 72.39,80.01 58.42,80.01 R33.P$1 49.53,80.01 | 72.39,80.01 U3.14 | R19.P$2 73.03,86.36 72.39,85.72 72.39,80.01
+12V  (via drill 0.9)
  Top 0.406: v17.78,45.72 17.78,46.35 16.51,47.62 16.51,57.78 17.78,59.05 v17.78,60.96
  Bottom 0.406: R1.P$2 20.95,42.55 v17.78,45.72 | 16.19,78.42 17.78,76.83 v17.78,60.96
  Bottom 1.27: P1.DC+ 18.02,80.25 16.19,78.42 14.61,76.83 7.62,76.83 2.54,81.92 2.54,90.81 3.81,92.08 C1.+ 5.71,93.34 8.26,95.89 IC1.1
+UB
  Bottom 0.61: TB1.1 5.71,45.72 6.35,45.09 JP1.2
  Bottom 1.27: P1.AC1 2.71,53.51 1.78,52.32 1.78,46.61 2.54,45.72 TB1.1
-RESET
  Bottom 0.406: R47.P$1 U$1.37 34.29,36.2 33.66,35.56 R46.P$2
AIN-IAC
  Bottom 0.305: J-AN.3 U$1.31
AIN-IBAT
  Bottom 0.254: R32.P$1 34.92,21.59 40.01,26.67 40.01,30.48 40.64,31.11 43.18,31.11 44.45,32.38 44.45,41.27 42.55,42.55 41.27,42.55 40.01,41.27 40.01,38.73 38.73,37.47 35.56,37.47 34.92,38.1 34.92,43.81
  Bottom 0.305: C12.1 33.66,43.18 34.29,43.81 34.92,43.81 U$1.34
  Bottom 0.406: R31.P$1 R32.P$1
AIN-THERM1
  Bottom 0.406: R26.P$1 43.81,53.34 43.18,53.98 U$1.30
AIN-THERM2
  Bottom 0.406: R29.P$1 46.99,55.24 45.72,56.52 U$1.29
AIN-VAC
  Bottom 0.305: J-AN.2 U$1.32
AIN-VBAT
  Bottom 0.305: C9.+ 24.77,67.31 25.4,66.67 R24.P$1 25.4,59.05 26.04,58.42 C8.1 33.02,58.42 33.66,57.78 33.66,53.34 34.29,52.7 38.73,52.7 39.37,52.07 39.37,47.62 38.1,46.35 U$1.33
GND
  Top 0.61: R30.P$2 72.39,2.54 71.12,3.81 65.41,3.81 63.5,1.91 R27.P$2 60.33,3.81 55.88,8.26 41.91,8.26 | T2.1 T3.1 17.78,31.75 17.78,36.2 R2.P$1 | 41.91,8.26 34.92,8.26 | 34.92,8.26 R32.P$2 | J-AN2.3 41.91,8.26 | 34.92,8.26 26.04,8.26 20.32,2.54 8.26,2.54 4.45,6.35 2.79,6.35 1.52,7.62 1.4,46.48 TB1.2 | O2.2 18.41,95.25 | C10.2 48.26,19.68 | P1.AC2 7.79,62.53 7.87,62.61
  Bottom 0.61: LD1.K R30.P$2
  Bottom 1.27: P1.DC0V 7.86,82.31 5.71,84.45 C1.- | TB1.2 4.45,51.27 P1.AC2
  pour Top (isolate 0.61): 21.59,99.06 91.44,99.06 92.71,97.79 92.71,92.71 92.08,92.08 74.93,92.08 71.12,88.27 57.78,88.27 52.7,93.34 22.23,93.34 20.95,94.61 20.95,98.42
  pour Top (isolate 0.61): 0.64,62.23 0.64,99.06 19.05,99.06 19.68,98.42 19.68,93.34 20.95,92.08 51.44,92.08 56.52,87 71.75,87 75.56,90.81 83.82,90.81 85.09,89.53 85.09,11.43 84.45,10.79 22.86,10.79 21.59,12.06 21.59,20.95 17.78,24.77 17.78,43.18 18.41,46.35 18.41,61.59 1.27,61.59
INP-OFF  (via drill 0.9)
  Top 0.406: O2.4 v33.66,82.55
  Bottom 0.406: v33.66,82.55 33.66,81.92 33.02,81.92 29.84,78.74 28.57,78.74 27.94,78.11 27.94,75.56 29.84,73.66 R36.P$2 32.38,69.22 U$1.24 | C14.1 O2.4
INP-ON  (via drill 0.9)
  Top 0.406: O1.4 47.62,88.9 v41.27,82.55
  Bottom 0.406: v41.27,82.55 36.2,82.55 33.02,79.38 33.02,76.83 | 33.02,76.83 R34.P$2 U$1.23 | C13.+ 33.02,76.83
INP-SYNC  (via drill 0.9)
  Top 0.406: v47.62,85.09 45.72,85.09 43.18,82.55 43.18,81.28 42.55,80.64 v42.55,73.03
  Bottom 0.305: U$1.26 38.1,64.14 39.37,65.41 39.37,67.94 42.55,71.12 v42.55,73.03
  Bottom 0.406: OK1.6 60.33,94.61 60.96,93.98 R38.P$2
  Bottom 0.61: OK1.6 57.15,94.61 55.88,93.34 55.88,88.9 53.34,86.36 48.9,86.36 v47.62,85.09
LARGE-L
  Bottom 0.305: U5.1 64.14,38.73 59.69,34.29 56.52,34.29 54.61,32.38 53.34,31.11 U$1.2
LARGE-R
  Bottom 0.305: U5.11 70.48,31.11 69.22,32.38 63.5,32.38 62.23,33.66 57.15,33.66 55.24,31.75 55.24,31.11 U$1.1
LED
  Bottom 0.254: U3.1 64.14,78.11 62.87,77.47 62.87,75.56 61.59,74.3 61.59,73.03 59.05,70.48 48.26,70.48 44.45,74.3 U$1.22
MED-L
  Bottom 0.305: U$1.4 55.24,36.2 55.88,35.56 58.42,35.56 59.69,36.83 59.69,47.62 60.33,48.26 U4.5
MED-R
  Bottom 0.305: U$1.3 54.61,33.66 55.88,34.92 59.05,34.92 60.33,36.2 60.33,46.35 60.96,46.99 68.58,46.99 69.22,47.62 69.22,48.26 71.75,50.8 U4.11
N$1
  Bottom 0.305: U$1.10 J1.2
N$2
  Bottom 0.305: J1.3 U$1.11
N$3
  Bottom 0.305: J1.4 U$1.12
N$4
  Bottom 0.305: J1.5 U$1.13
N$5
  Bottom 0.406: U2.1 26.67,25.4 22.86,29.21 22.86,32.38 22.23,33.02 U2.5
N$6
  Bottom 0.406: U2.4 27.94,34.92 R2.P$2 29.21,38.1 R1.P$1
N$7
  Bottom 0.305: BI-LED.2 92.08,90.81 R20.P$2 R19.P$1
N$8
  Bottom 0.254: U3.2 66.67,75.56 66.93,75.31 69.6,75.31 71.12,76.83 73.66,76.83 75.56,78.74
  Bottom 0.305: 75.56,78.74 75.56,79.38 74.3,80.64 74.3,81.92 75.56,83.19 90.17,83.19 BI-LED.1
N$14
  Bottom 0.61: JP1.3 R21.P$2
N$15
  Bottom 0.254: R3.P$1 78.11,81.28 78.74,80.64 78.74,76.83 77.47,75.56 76.2,75.56 74.93,74.3 74.93,73.66 74.3,73.03 U3.12 68.58,69.22 62.87,69.22 62.87,71.75 64.14,73.03 U3.3
N$16
  Bottom 0.254: U3.4 67.44,73.28 69.85,73.28 70.87,74.3 73.66,74.3 74.93,75.56 74.93,76.83 75.56,77.47 R4.P$1
N$17
  Bottom 0.254: U3.6 67.44,65.41 71.25,69.22
  Bottom 0.305: 71.25,69.22 74.93,69.22 | 74.93,69.22 74.93,71.75 R5.P$1 | U3.9 74.3,65.41 74.93,66.04 74.93,69.22
N$18
  Bottom 0.305: U3.8 73.03,62.87 76.83,66.67 R6.P$1
N$19
  Bottom 0.254: U3.10 72.26,67.94 70.23,65.91 70.23,61.72 70.1,61.59
  Bottom 0.305: U4.1 67.31,58.42 67.94,59.05 67.94,60.96 68.58,61.59 70.1,61.59 74.3,61.59 R7.P$1
N$20
  Bottom 0.305: U4.2 66.67,55.88 71.12,60.33 R8.P$1
N$21
  Bottom 0.305: U4.3 U4.12 73.66,53.34 R9.P$1
N$22
  Bottom 0.305: U4.4 66.04,50.8 67.31,52.07 74.3,52.07 74.93,52.7 R10.P$1
N$23
  Bottom 0.406: R11.P$1 75.56,46.99 74.3,45.72 U4.9 U4.6
N$24
  Bottom 0.406: U4.8 R12.P$1
N$25
  Bottom 0.406: U5.13 73.66,36.2 R13.P$1 78.74,41.27 78.74,47.62 77.47,48.9 75.56,48.9 74.93,48.26 U4.10
N$26
  Bottom 0.406: U5.12 74.93,33.66 R14.P$1
N$27
  Top 0.305: U5.3 U5.2
  Bottom 0.305: U5.3 69.22,33.66 70.48,32.38 76.2,32.38 76.83,31.75 R15.P$1
N$28
  Bottom 0.305: R16.P$1 76.2,26.04 74.93,27.3 68.58,27.3 U5.4
N$29
  Top 0.305: U5.9 U5.10
  Bottom 0.305: U5.9 73.03,26.04 R17.P$1
N$30
  Bottom 0.305: U5.8 72.39,22.86 R18.P$1
N$32
  Top 0.61: JP1.1 3.81,41.91 5.08,43.18 13.34,43.18 14.61,41.91 R22.P$2
N$34
  Bottom 0.254: 18.41,49.53 19.05,48.9 20.32,48.9 20.95,49.53 22.23,49.53 22.86,48.9 R40.E
  Bottom 0.406: R21.P$1 R22.P$1 16.51,51.44 18.41,49.53
N$35
  Bottom 0.406: R27.P$1 R25.P$2 C10.1 53.34,19.05 45.72,26.67 45.72,41.27 45.09,41.91 R26.P$2
N$36
  Bottom 0.61: J4.2 63.5,5.08 66.67,1.91 R28.P$1
N$37
  Top 0.61: J3.2 51.44,3.17 52.7,1.91 R25.P$1
N$38
  Bottom 0.254: R29.P$2 47.62,43.18 46.35,41.91 46.35,27.3 58.42,15.24 60.96,15.24 64.14,12.06 C11.1
  Bottom 0.406: R30.P$1 R28.P$2 67.94,12.06 66.04,10.16 C11.1
N$39
  Bottom 0.61: R33.P$2 51.44,91.44 J-SWON.1
N$40
  Bottom 0.61: TB2.11 89.53,81.28 R3.P$2
N$41
  Top 0.61: R31.P$2 42.55,1.91 44.45,3.81 J-AN2.2
N$42
  Bottom 0.61: O1.1 52.07,97.79 53.98,95.89 J-SWON.2
N$43
  Bottom 0.61: J-SYNCIN.1 85.09,93.34 R37.P$1
N$44
  Bottom 0.61: J-SYNCIN.2 88.9,96.52 88.27,97.16 D1.A 74.93,97.16 73.28,98.81 70.23,98.81 69.85,98.42 69.85,96.52 67.94,94.61 OK1.3
N$45
  Bottom 0.61: R35.P$2 36.83,97.79 37.47,97.16 J-SWOFF.1
N$46
  Bottom 0.61: O2.1 33.66,93.98 35.56,92.08 39.37,92.08 40.01,92.71 J-SWOFF.2
N$47
  Bottom 0.61: D1.C R37.P$2 70.48,92.08 OK1.2
N$49
  Bottom 0.406: LD1.A 76.83,5.71 78.11,6.99 O3.2
N$50
  Bottom 0.406: O3.1 78.11,12.7 80.64,15.24 R39.P$1
N$51
  Bottom 0.406: R42.P$2 18.41,19.68 15.24,22.86 15.24,26.04 12.7,28.57 5.71,28.57 4.45,29.84 4.45,32.38 5.08,33.02 T2.3
  Bottom 0.61: Q1.G 16.51,13.97 18.41,15.88 R42.P$2
N$52
  Top 0.813: O3.3 85.72,8.89 87.63,6.99 95.89,6.99 96.52,7.62 96.52,9.27 Q3.B
N$53
  Bottom 0.254: R41.P$1 43.81,38.73 43.81,33.02 43.18,32.38 34.92,32.38 34.92,24.77 32.38,22.23 19.05,22.23 16.51,24.77 16.51,27.3 13.97,29.84 9.53,29.84
  Bottom 0.406: 9.53,29.84 6.99,29.84 5.71,31.11 5.71,32.38 T2.2
N$54
  Top 1.27: Q2.S 7.62,20.32 6.99,19.68 6.99,16.51 TB-FAN.1
  Bottom 0.61: Q1.S 11.43,8.89 12.06,8.26 R44.P$1 R42.P$1
  Bottom 1.27: TB-FAN.1 3.81,8.89 Q1.S
N$55
  Bottom 0.406: T3.3 9.53,36.2 4.45,36.2 3.17,34.92 3.17,27.94 3.81,27.3 5.71,27.3 7.62,25.4 Q2.G
  Bottom 0.61: R44.P$2 13.34,20.32 13.34,24.77 12.7,25.4 Q2.G
N$56
  Bottom 0.305: U5.6 66.04,26.04 R45.P$2
N$57
  Bottom 1.27: TB-FAN.2 5.08,17.14 6.35,15.88 6.35,12.7 7.62,11.43 Q1.D
N$58
  Bottom 0.406: R43.P$1 12.7,38.1 13.34,37.47 13.34,36.2 13.97,35.56 T3.2
N$59
  Bottom 0.406: J-50HZ.1 61.59,20.32 R45.P$1
N$60
  Bottom 1.27: TB-FAN.3 4.45,20.95 6.35,22.86 Q2.D
N$62
  Bottom 0.61: R4.P$2 87.63,77.47 88.9,76.2 TB2.12
N$63
  Bottom 0.61: R5.P$2 TB2.13
N$64
  Bottom 0.61: R6.P$2 88.27,69.85 89.53,71.12 TB2.14
N$65
  Bottom 0.61: TB3.11 89.53,64.14 R7.P$2
N$66
  Bottom 0.61: R8.P$2 88.9,60.33 90.17,59.05 TB3.12
N$67
  Bottom 0.61: R9.P$2 TB3.13
N$68
  Bottom 0.61: R10.P$2 89.53,52.7 90.81,53.98 TB3.14
N$69
  Bottom 0.61: R11.P$2 89.53,46.99 TB4.11
N$70
  Bottom 0.61: R12.P$2 88.27,43.18 89.53,41.91 TB4.12
N$71
  Bottom 0.61: R13.P$2 TB4.13
N$72
  Bottom 0.61: R14.P$2 87.63,35.56 88.9,36.83 TB4.14
N$73
  Bottom 0.61: R15.P$2 89.53,29.84 TB5.11
N$74
  Bottom 0.61: R16.P$2 88.27,26.04 89.53,24.77 TB5.12
N$75
  Bottom 0.61: R17.P$2 TB5.13
N$76
  Bottom 0.61: R18.P$2 88.9,18.41 90.17,19.68 TB5.14
N$77
  Bottom 0.406: U2.7 22.23,27.94 26.67,23.5 29.84,23.5 R46.P$1
N$78
  Top 0.813: TB-RELAY.2 85.72,5.71 83.82,7.62 83.82,10.16 O3.4
  Bottom 0.813: Q3.C 93.98,12.06 93.34,12.7 D2.A 86.36,12.7 O3.4
N$79
  Bottom 0.813: TB-RELAY.1 92.08,6.35 97.79,6.35 98.42,7.24 D2.C
N$81
  Bottom 0.813: Q3.E 89.53,9.53 87,6.99 85.09,6.99 TB-RELAY.3
N$82
  Bottom 0.406: R40.S 25.4,48.26 26.67,49.53 26.67,52.07 R24.P$2 24.77,52.7 24.13,52.7 22.23,50.8 C7.1
N$84
  Bottom 0.406: R23.P$2 24.13,55.24 29.21,55.24 29.84,54.61 29.84,50.8 27.94,48.9 R40.A
OP-50HZ  (via drill 0.9)
  Top 0.305: v47.62,40.64 47.62,41.91 46.99,42.55 46.99,43.18 45.72,45.09 45.72,47.62 v47.62,49.53 | v40.64,66.67 U$1.25
  Bottom 0.254: v47.62,49.53 48.9,49.53 49.53,50.16 49.53,53.34 50.16,53.98 50.16,57.15 45.72,61.59
  Bottom 0.305: U5.5 63.5,28.57 62.87,29.21 62.87,31.75 61.59,33.02 57.78,33.02 55.88,31.11 55.88,30.48 54.61,29.21 54.61,27.94 53.34,26.67 51.44,26.67 50.8,27.3 50.8,30.48 49.53,31.75 49.53,35.56 47.62,37.47 v47.62,40.64 | 45.72,61.59 v40.64,66.67
OP-SYNCED  (via drill 0.9)
  Top 0.305: U$1.5 54.61,38.73 55.24,38.1 55.24,34.29 v58.42,31.11
  Bottom 0.305: v58.42,31.11 59.69,29.84 59.69,25.4 63.5,21.59 67.31,21.59 69.85,19.05 70.48,19.05 72.39,17.14 74.93,17.14 R39.P$2
PWM-FAN1
  Bottom 0.254: 40.01,58.42 47.62,58.42 49.53,56.52 49.53,54.61 48.26,53.34 48.26,51.44 47.62,50.8 R41.P$2
  Bottom 0.305: U$1.28 39.37,59.05 40.01,58.42
PWM-FAN2  (via drill 0.9)
  Top 0.254: v17.78,55.24 17.78,50.16 v19.68,47.62
  Bottom 0.254: 27.94,62.87 27.94,69.22 25.4,71.75 20.32,71.75 19.05,70.48 19.05,56.52 v17.78,55.24 | v19.68,47.62 18.41,47.62 17.78,48.26 16.51,48.26 15.88,47.62 15.88,45.09 17.14,43.81 17.14,40.64 15.88,39.37 R43.P$2
  Bottom 0.305: U$1.27 36.2,61.59 34.29,63.5 28.57,63.5 27.94,62.87
RX1
  Bottom 0.305: J2.2 56.52,42.55 55.24,43.81 U$1.7
SMALL-L
  Bottom 0.254: 71.5,70.48 67.69,66.67 62.23,66.67 | U$1.35 44.45,48.26 49.53,48.26 50.16,48.9 50.16,52.7 50.8,53.34 50.8,65.41
  Bottom 0.305: U3.11 71.5,70.48 | 50.8,65.41 60.96,65.41 62.23,66.67
SMALL-R
  Bottom 0.254: U$1.36 38.1,38.73 39.37,40.01 39.37,41.91 45.09,47.62 50.16,47.62 50.8,48.26 50.8,52.07 51.44,52.7
  Bottom 0.305: U4.13 71.75,55.88 69.85,53.98 67.31,53.98 66.67,54.61 62.23,54.61 60.33,52.7 51.44,52.7
TINY-L
  Bottom 0.254: U3.13 70.99,75.56 69.72,74.3 63.88,74.3 58.8,69.22 U$1.17
TINY-R
  Bottom 0.254: U3.5 56.52,67.94 55.24,66.67 U$1.16
TX1
  Bottom 0.305: J2.3 56.52,40.01 55.24,41.27 U$1.6

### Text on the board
tPlace: Tiny | Small | -B | +B | 48v | Medium | Mack-e- | - | Large | F2 | stm32 WarpVerter | 201904 | F1 | + | - | -RLY | + | Therm1 | Therm2 | Syncd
